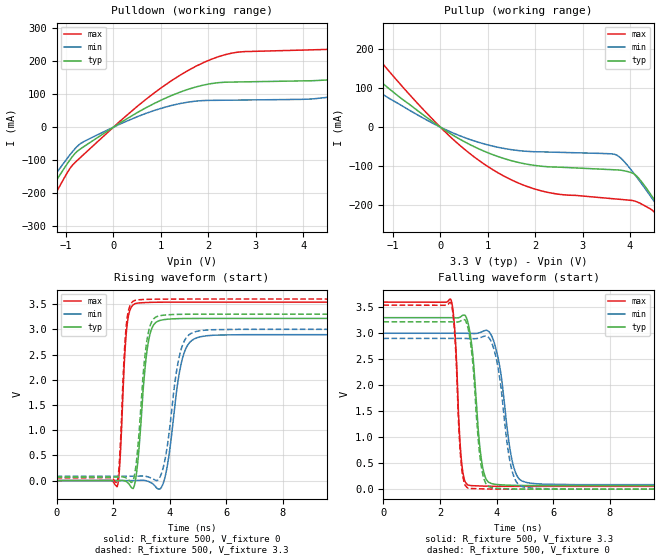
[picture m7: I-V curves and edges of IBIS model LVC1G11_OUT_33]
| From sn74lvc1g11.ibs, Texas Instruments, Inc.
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[Model]   LVC1G11_OUT_33
Model_type  Output
Vref =   0
Rref =   500
Cref =   50p
Vmeas =   1.5
| variable   typ   min   max
C_comp   8.37pF   6.24pF   10.52pF
| C_pullup   8.48pF   6.24pF   9.73pF
| C_pulldown   8.25pF   6.33pF   10.52pF
[Temperature Range]   40   100   -40
| Ambient temperature   25   85   -40
[Voltage range]   3.3   3   3.6
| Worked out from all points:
|   slope of the pulldown table from 0 to 0.495 V, typ, clamps not added: 11.3 ohm
|   slope of the pullup table from 0 to 0.495 V, typ, clamps not added: 13.5 ohm
|   rising waveform, R_fixture 500, V_fixture 0: 20-80 % time 282ps typ, 411ps min, 180ps max; typ from 0 V to 3.22 V
|   falling waveform, R_fixture 500, V_fixture 3.3: 20-80 % time 283ps typ, 415ps min, 182ps max; typ from 3.3 V to 0.069 V
|   rising waveform, R_fixture 500, V_fixture 3.3: 20-80 % time 281ps typ, 413ps min, 178ps max; typ from 0.069 V to 3.3 V
|   falling waveform, R_fixture 500, V_fixture 0: 20-80 % time 277ps typ, 400ps min, 179ps max; typ from 3.22 V to 0 V
[Pulldown]
| LVC1G11_OUT_33
|   Voltage   I(typ)   I(min)   I(max)
-5.5V     -1.112A    -993.8mA   -1.301A
-2.095V   -365.2mA   -321.2mA   -435.6mA
-1.48V    -224.6mA   -195.7mA   -271.3mA
-705mV    -67mA      -50.96mA   -93.4mA
1.895V    127.7mA    80.8mA     195.8mA
4.735V    148.3mA    96.37mA    238.3mA
6.005V    208mA      150.5mA    305.3mA
6.98V     278.7mA    201.6mA    397mA
7.35V     308.5mA    129.4mA    437.6mA
7.84V     330.1mA    92.52mA    494.8mA
8.75V     170.8mA    93.27mA    501.3mA
11V       160mA      96.49mA    277.5mA
[Pullup]
| LVC1G11_OUT_33
|   Voltage   I(typ)   I(min)   I(max)
-5.5V     620.3mA    489.5mA    867.8mA
-3.245V   338.6mA    262.4mA    480.1mA
-2.5V     251.3mA    193mA      358.8mA
-1.96V    190.8mA    145.3mA    273.9mA
-50mV     4.153mA    3.023mA    6.162mA
1.115V    -70.96mA   -48.91mA   -109.6mA
2.135V    -100.3mA   -63.39mA   -163.5mA
3.715V    -109.6mA   -71.54mA   -184.3mA
4.15V     -126.7mA   -129.5mA   -191.7mA
4.79V     -237.7mA   -240mA     -270mA
4.985V    -275.2mA   -275.3mA   -310.9mA
11V       -1.523A    -1.428A    -1.714A
[Ramp]
| LVC1G11_OUT_33
| variable   typ   min   max
dV/dt_r   2.02/3.06E-10   1.84/4.40E-10   2.20/1.89E-10
dV/dt_f   1.97/2.96E-10   1.78/4.34E-10   2.16/1.90E-10
R_load = 500
[Rising Waveform]
| LVC1G11_OUT_33
R_fixture =   500
C_fixture =   0
L_fixture =   0
V_fixture =   0
V_fixture_min = 0
V_fixture_max = 0
|   Time   V(typ)   V(min)   V(max)
0s        141.8pV    4.978nV    2.433nV
2.145ns   269.3uV    5.445uV    -122.9mV
2.245ns   2.184mV    -30.65uV   380.4mV
2.485ns   -26.09mV   -151.7uV   3.018V
2.81ns    58.7mV     1.076mV    3.514V
3.235ns   2.695V     -13.45mV   3.533V
3.715ns   3.183V     -130.5mV   3.538V
4.455ns   3.213V     2.418V     3.539V
5.105ns   3.216V     2.854V     3.539V
28.99ns   3.216V     2.894V     3.539V
[Falling Waveform]
| LVC1G11_OUT_33
R_fixture =   500
C_fixture =   0
L_fixture =   0
V_fixture =   3.3
V_fixture_min = 3
V_fixture_max = 3.6
|   Time   V(typ)   V(min)   V(max)
0s        3.3V       3V         3.6V
2.39ns    3.3V       3V         3.644V
2.535ns   3.297V     3V         2.976V
2.75ns    3.323V     3V         606.4mV
3ns       3.183V     2.998V     77.67mV
3.48ns    516.4mV    3.027V     60.28mV
3.885ns   99.61mV    2.872V     55.96mV
4.575ns   74.07mV    493.4mV    54.36mV
5.09ns    70.67mV    124.6mV    54.11mV
28.99ns   69.38mV    85.91mV    53.96mV
[Rising Waveform]
| LVC1G11_OUT_33
R_fixture =   500
C_fixture =   0
L_fixture =   0
V_fixture =   3.3
V_fixture_min = 3
V_fixture_max = 3.6
|   Time   V(typ)   V(min)   V(max)
0s        69.35mV    85.87mV    53.95mV
2.145ns   69.62mV    85.88mV    -36.36mV
2.24ns    71.36mV    85.85mV    507.5mV
2.475ns   49.02mV    85.73mV    3.107V
2.805ns   266.2mV    86.9mV     3.578V
3.2ns     2.78V      79.06mV    3.594V
3.635ns   3.267V     43.75mV    3.599V
4.385ns   3.297V     2.552V     3.6V
4.99ns    3.3V       2.963V     3.6V
28.99ns   3.3V       3V         3.6V
[Falling Waveform]
| LVC1G11_OUT_33
R_fixture =   500
C_fixture =   0
L_fixture =   0
V_fixture =   0
V_fixture_min = 0
V_fixture_max = 0
|   Time   V(typ)   V(min)   V(max)
0s        3.22V      2.9V       3.542V
2.385ns   3.22V      2.9V       3.585V
2.53ns    3.218V     2.9V       2.915V
2.745ns   3.241V     2.9V       526.6mV
2.99ns    3.104V     2.899V     21.09mV
3.45ns    477mV      2.92V      6.28mV
3.835ns   29.57mV    2.81V      2.11mV
4.515ns   4.786mV    429.1mV    436.5uV
5.005ns   1.417mV    37.27mV    176.8uV
28.99ns   24.43uV    28.97uV    18.76uV
